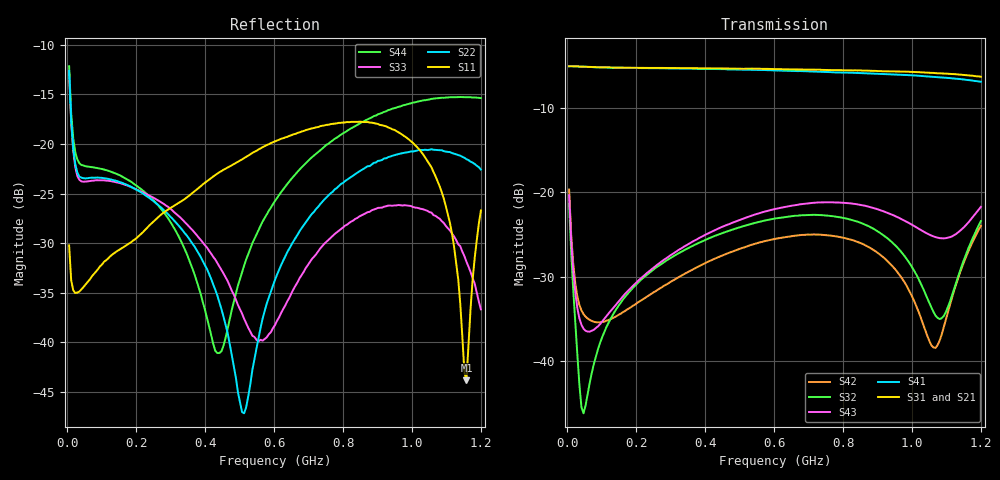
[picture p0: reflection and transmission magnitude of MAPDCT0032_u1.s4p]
#	MHz	S	dB	R	75
!FREQ	R1	I1	R2	I2	R3	I3	R4	I4
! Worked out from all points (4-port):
!   201 points, 5 MHz to 1.2 GHz, reference 75 ohm
!   strongest paths, dB at 5 MHz, 303.8 MHz, 602.5 MHz, 901.2 MHz, 1.2 GHz:
!     S31: -5.1, -5.3, -5.4, -5.7, -6.3
!     S41: -5.1, -5.4, -5.6, -6.0, -6.9
!     S21: -5.1, -5.4, -5.6, -5.9, -6.6
!     S43: -20.4, -27.3, -22.0, -22.0, -21.7
!     S32: -21.4, -27.7, -23.1, -24.6, -23.4
!     S42: -19.7, -30.5, -25.5, -27.2, -24.0
!   lowest |S11| = -43.8 dB at 1.158 GHz (marker M1), VSWR 1.01, Z = 75.9 + j0.286 ohm
!   |S11| at or under -10 dB: start of sweep to end of sweep
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5  -30.23 130.9  -5.09 0.6  -5.10 0.5  -5.10 0.5
   -5.09 0.5  -12.62 133.0  -21.50 -56.5  -19.73 -48.1
   -5.10 0.5  -21.41 -56.5  -12.91 132.9  -20.40 -47.9
   -5.09 0.5  -19.68 -47.7  -20.36 -47.7  -12.16 136.0
46.825  -34.43 164.0  -5.15 -5.7  -5.14 -6.0  -5.14 -6.0
        -5.15 -5.8  -23.46 159.8  -46.17 -8.6  -34.42 -24.8
        -5.15 -6.0  -46.15 -8.3  -23.81 159.3  -36.14 -17.6
        -5.15 -6.0  -34.42 -24.8  -36.14 -17.8  -22.17 159.7
435.2  -22.99 56.5  -5.45 -50.6  -5.35 -53.0  -5.44 -52.2
       -5.45 -50.6  -35.30 116.1  -25.03 46.3  -27.71 40.8
       -5.34 -53.0  -25.05 46.3  -32.01 108.4  -24.34 48.2
       -5.43 -52.3  -27.73 40.7  -24.36 48.2  -41.09 54.3
512.875  -21.43 39.7  -5.52 -60.0  -5.39 -62.8  -5.51 -61.9
         -5.51 -60.0  -47.17 31.6  -23.98 40.9  -26.51 37.7
         -5.40 -62.9  -23.99 40.9  -37.63 75.4  -23.07 44.1
         -5.51 -61.9  -26.53 37.7  -23.09 44.1  -32.27 -28.4
1002.825  -19.90 -57.3  -6.04 -129.0  -5.78 -134.0  -6.21 -130.2
          -6.02 -129.3  -20.76 -102.0  -29.04 3.1  -32.57 6.5
          -5.77 -134.2  -29.04 2.9  -26.36 -106.4  -23.95 19.5
          -6.18 -130.5  -32.55 6.2  -23.91 19.4  -15.83 -84.6
1158.175  -43.83 17.0  -6.42 -157.6  -6.17 -162.7  -6.75 -157.5
          -6.39 -157.8  -21.54 -121.8  -27.17 101.3  -27.52 112.6
          -6.14 -162.9  -27.21 101.2  -31.89 -144.1  -23.85 62.0
          -6.71 -157.8  -27.52 112.4  -23.83 61.7  -15.29 -93.8
1200  -26.71 68.7  -6.60 -166.2  -6.35 -171.3  -6.99 -165.5
      -6.57 -166.4  -22.59 -126.9  -23.40 101.7  -23.98 109.9
      -6.33 -171.4  -23.41 101.6  -36.68 -173.8  -21.77 69.7
      -6.93 -165.8  -23.97 109.7  -21.73 69.4  -15.37 -94.8
